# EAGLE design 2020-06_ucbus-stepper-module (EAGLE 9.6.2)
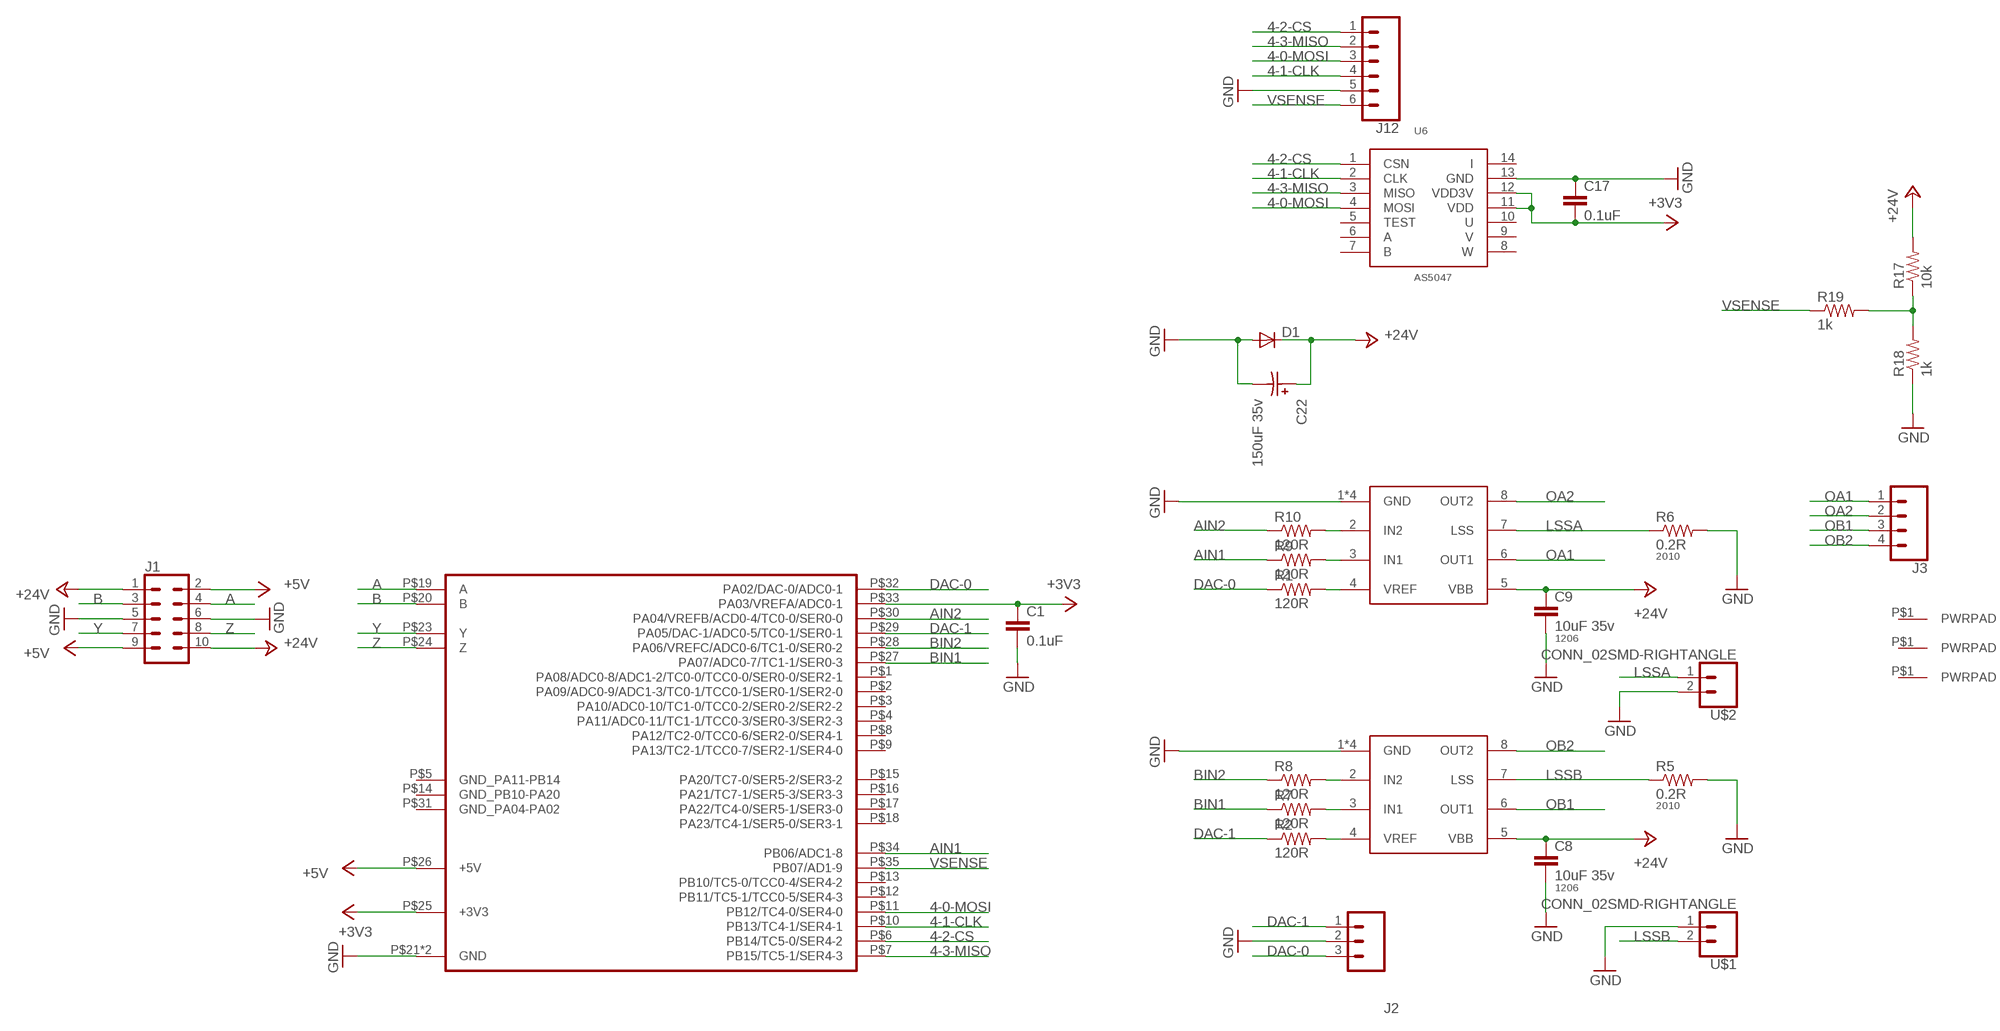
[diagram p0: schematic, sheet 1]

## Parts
C1  0.1uF  CAP0805  [0805]
C8  10uF 35v  CAP1206  [1206]
C9  10uF 35v  CAP1206  [1206]
C17  0.1uF  CAP0805  [0805]
C22  150uF 35v  CAP-POLCAP_POL_SMD6.6X6.6  [SMD-ELEC-CAP]
D1  DIODESMA403D  [SMA-403D]
J1  CONN_05X2SHD_LOCK  [2X5-SHROUDED_LOCK]
J2  CONN_03SMD_RA_MALE  [1X03_SMD_RA_MALE]
J3  CONN_04SCREW_LOCK  [SCREWTERMINAL-3.5MM-4_LOCK]
J4  PWRPADM3-SKINNY  [PWRPAD_3-25MM-SKINNY]
J5  PWRPADM3-SKINNY  [PWRPAD_3-25MM-SKINNY]
J6  PWRPADM3-SKINNY  [PWRPAD_3-25MM-SKINNY]
J12  CONN_06SMD-FEMALE-V2  [1X06-SMD-FEMALE]
R1  120R  RESISTOR0805-RES  [0805]
R2  120R  RESISTOR0805-RES  [0805]
R5  0.2R  RESISTOR2010  [R2010]
R6  0.2R  RESISTOR2010  [R2010]
R7  120R  RESISTOR0805-RES  [0805]
R8  120R  RESISTOR0805-RES  [0805]
R9  120R  RESISTOR0805-RES  [0805]
R10  120R  RESISTOR0805-RES  [0805]
R17  10k  RESISTOR0805-RES  [0805]
R18  1k  RESISTOR0805-RES  [0805]
R19  1k  RESISTOR0805-RES  [0805]
U1  UCBUS_MODULE  [UCBUS_MODULE]
U2  A4950THRU  [SOIC8_PAD_THRU]
U3  A4950THRU  [SOIC8_PAD_THRU]
U6  AS5047  [TSSOP14]
U$1  CONN_02SMD-RIGHTANGLE  [1X02_SMD_RA_MALE]
U$2  CONN_02SMD-RIGHTANGLE  [1X02_SMD_RA_MALE]

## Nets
4-0-MOSI: J12.3 U1.P$11(PB12/TC4-0/SER4-0) U6.4(MOSI)
4-1-CLK: J12.4 U1.P$10(PB13/TC4-1/SER4-1) U6.2(CLK)
4-2-CS: J12.1 U1.P$6(PB14/TC5-0/SER4-2) U6.1(CSN)
4-3-MISO: J12.2 U1.P$7(PB15/TC5-1/SER4-3) U6.3(MISO)
+3V3: C1.1 C17.2 U1.P$25(+3V3) U1.P$33(PA03/VREFA/ADC0-1) U6.11(VDD) U6.12(VDD3V)
+5V: J1.2 J1.9 U1.P$26(+5V)
+24V: C8.1 C9.1 C22.A D1.P$1(C) J1.1 J1.10 R17.2 U2.5(VBB) U3.5(VBB)
A: J1.4 U1.P$19(A)
AIN1: R9.1 U1.P$34(PB06/ADC1-8)
AIN2: R10.1 U1.P$30(PA04/VREFB/ACD0-4/TC0-0/SER0-0)
B: J1.3 U1.P$20(B)
BIN1: R7.1 U1.P$27(PA07/ADC0-7/TC1-1/SER0-3)
BIN2: R8.1 U1.P$28(PA06/VREFC/ADC0-6/TC1-0/SER0-2)
DAC-0: J2.3 R1.1 U1.P$32(PA02/DAC-0/ADC0-1)
DAC-1: J2.1 R2.1 U1.P$29(PA05/DAC-1/ADC0-5/TC0-1/SER0-1)
GND: C1.2 C8.2 C9.2 C17.1 C22.C D1.P$2(A) J1.5 J1.6 J2.2 J12.5 R5.2 R6.2 R18.1 U1.P$21(GND) U1.P$22(GND) U2.1(GND) U2.P$1(GND) U2.P$2(GND) U2.P$3(GND) U3.1(GND) U3.P$1(GND) U3.P$2(GND) U3.P$3(GND) U6.13(GND) U$1.1 U$2.2
LSSA: R6.1 U3.7(LSS) U$2.1
LSSB: R5.1 U2.7(LSS) U$1.2
N$1: R9.2 U3.3(IN1)
N$2: R2.2 U2.4(VREF)
N$3: R1.2 U3.4(VREF)
N$4: R10.2 U3.2(IN2)
N$7: R8.2 U2.2(IN2)
N$8: R7.2 U2.3(IN1)
N$17: R17.1 R18.2 R19.2
OA1: J3.1 U3.6(OUT1)
OA2: J3.2 U3.8(OUT2)
OB1: J3.3 U2.6(OUT1)
OB2: J3.4 U2.8(OUT2)
VSENSE: J12.6 R19.1 U1.P$35(PB07/AD1-9)
Y: J1.7 U1.P$23(Y)
Z: J1.8 U1.P$24(Z)
Unconnected: J4.P$1(PWRPAD) J5.P$1(PWRPAD) J6.P$1(PWRPAD) U1.P$1(PA08/ADC0-8/ADC1-2/TC0-0/TCC0-0/SER0-0/SER2-1) U1.P$2(PA09/ADC0-9/ADC1-3/TC0-1/TCC0-1/SER0-1/SER2-0) U1.P$3(PA10/ADC0-10/TC1-0/TCC0-2/SER0-2/SER2-2) U1.P$4(PA11/ADC0-11/TC1-1/TCC0-3/SER0-3/SER2-3) U1.P$5(GND_PA11-PB14) U1.P$8(PA12/TC2-0/TCC0-6/SER2-0/SER4-1) U1.P$9(PA13/TC2-1/TCC0-7/SER2-1/SER4-0) U1.P$12(PB11/TC5-1/TCC0-5/SER4-3) U1.P$13(PB10/TC5-0/TCC0-4/SER4-2) U1.P$14(GND_PB10-PA20) U1.P$15(PA20/TC7-0/SER5-2/SER3-2) U1.P$16(PA21/TC7-1/SER5-3/SER3-3) U1.P$17(PA22/TC4-0/SER5-1/SER3-0) U1.P$18(PA23/TC4-1/SER5-0/SER3-1) U1.P$31(GND_PA04-PA02) U6.5(TEST) U6.6(A) U6.7(B) U6.8(W) U6.9(V) U6.10(U) U6.14(I)

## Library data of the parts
C1 C17 = passives:CAP: Capacitor; PACKAGE: 0805
C8 C9 = passives:CAP: Capacitor; PACKAGE: 1206
C22 = passives:CAP-POL
D1 = passives:DIODE: DIODE
J1 = SparkFun-Connectors:CONN_05X2: Multi connection point. Often used as Generic Header-pin footprint for 0.1 inch spaced/style header connections For AVR SPI programming port, see special device with nice symbol: "AVR_SPI_PROG_5x2.dev" You can populate with any combo of single row headers, but if you'd like an exact match, check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; PROD_ID: CONN-08671; SF_ID: PRT-08506
J2 = SparkFun-Connectors:CONN_03: Multi connection point. Often used as Generic Header-pin footprint for 0.1 inch spaced/style header connections On any of the 0.1 inch spaced packages, you can populate with these: Break Away Headers - Straight (PRT-00116) Break Away Male Headers - Right Angle (PRT-00553) Female Headers (PRT-00115)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; PROD_ID: CONN-10925
J3 = SparkFun-Connectors:CONN_04: Multi connection point. Often used as Generic Header-pin footprint for 0.1 inch spaced/style header connections On any of the 0.1 inch spaced packages, you can populate with these: Break Away Headers - Straight (PRT-00116) Break Away Male Headers - Right Angle (PRT-00553) Female Headers (PRT-00115)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
J4-J6 = connector:PWRPAD
J12 = SparkFun-Connectors:CONN_06: Multi connection point. Often used as Generic Header-pin footprint for 0.1 inch spaced/style header connections On any of the 0.1 inch spaced packages, you can populate with these: Break Away Headers - Straight (PRT-00116) Break Away Male Headers - Right Angle (PRT-00553) Female Headers (PRT-00115)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; PROD_ID: CONN-09668
R1 R2 R7-R10 R17-R19 = passives:RESISTOR: Resistor; PACKAGE: 0805
R5 R6 = passives:RESISTOR: Resistor; PACKAGE: 2010
U1 = connector:UCBUS_MODULE
U2 U3 = power:A4950
U6 = sensor:AS5047
U$1 U$2 = connector:CONN_02

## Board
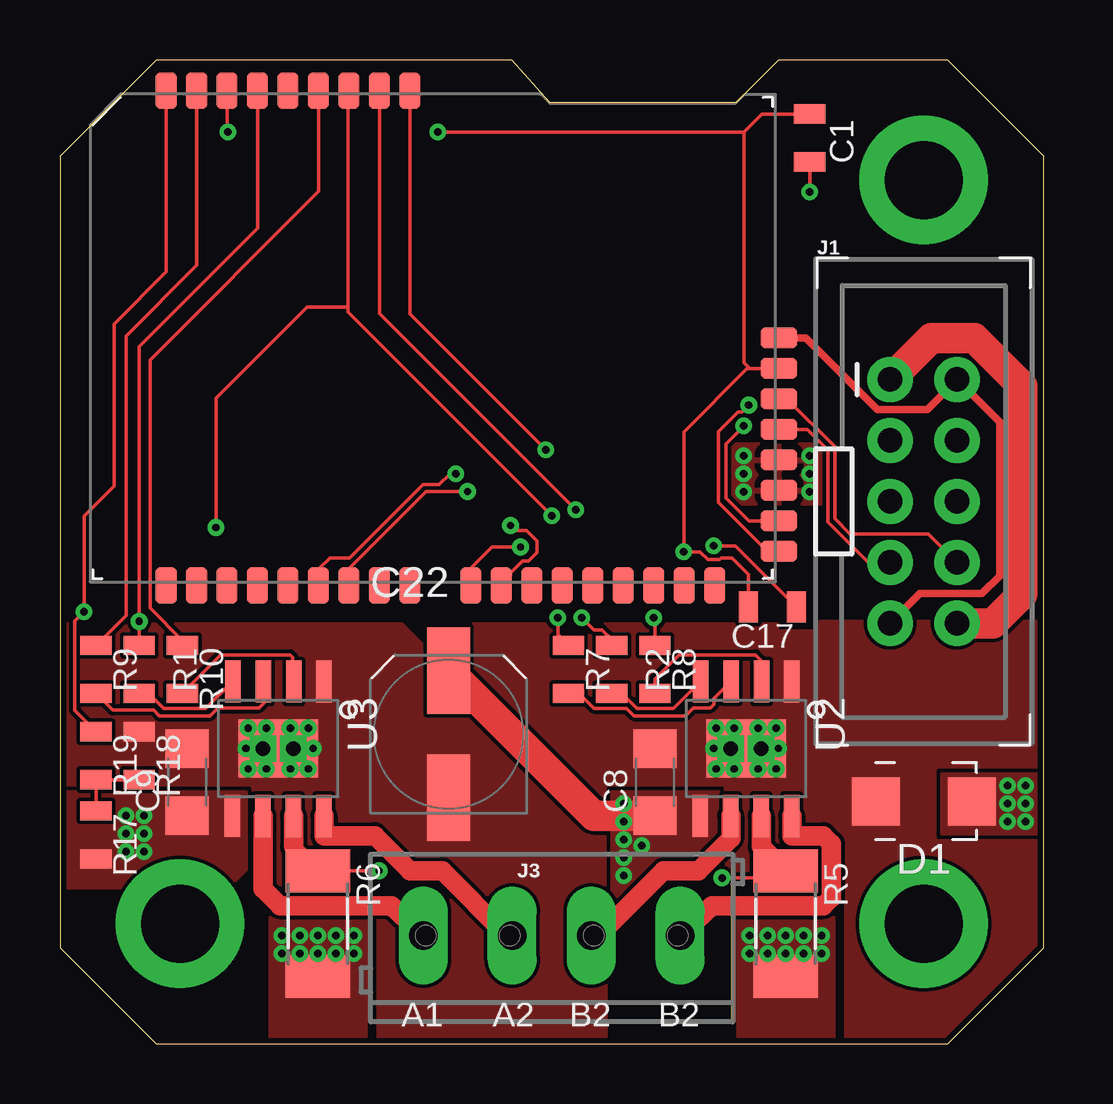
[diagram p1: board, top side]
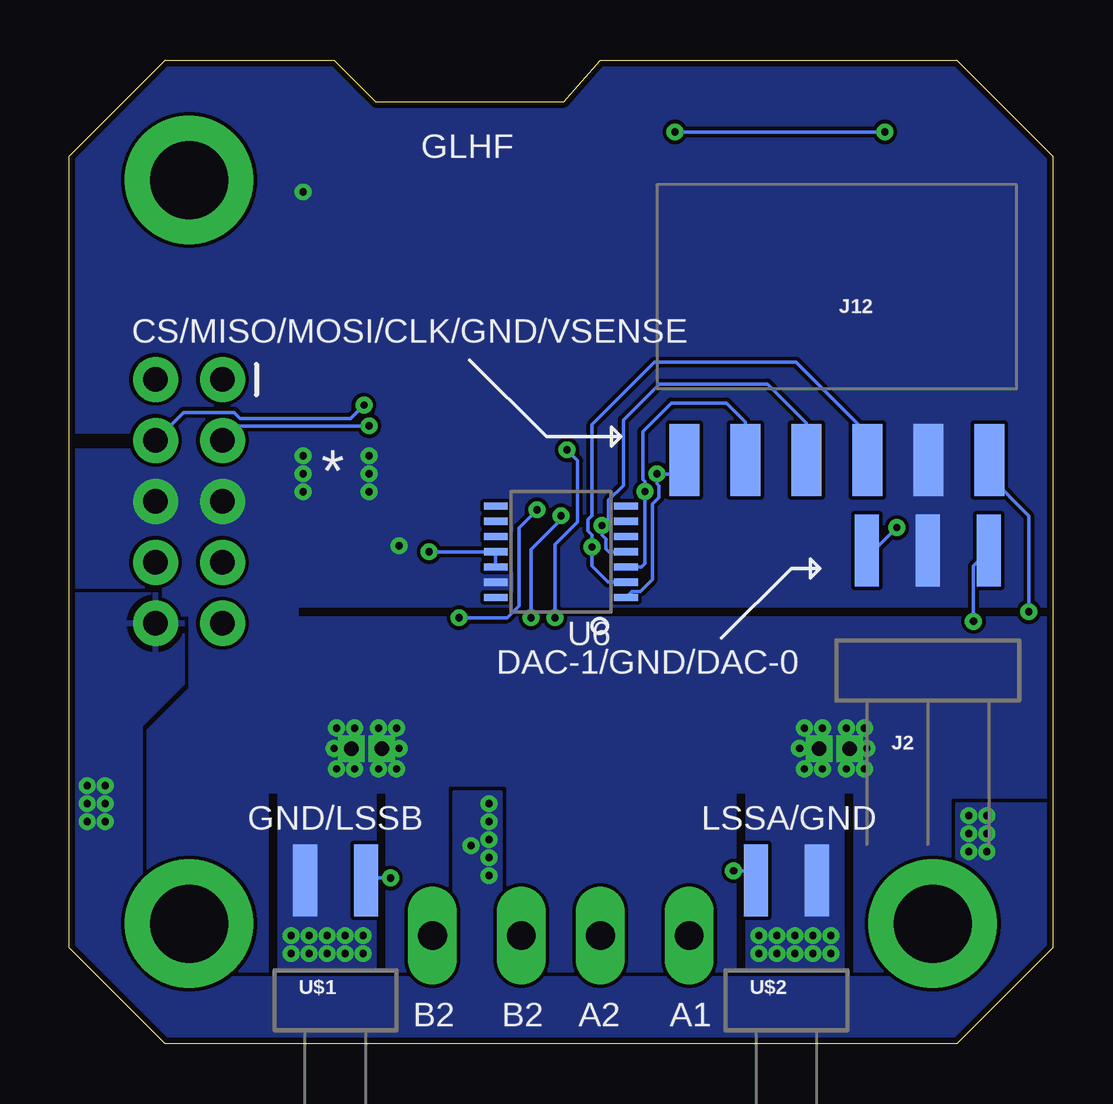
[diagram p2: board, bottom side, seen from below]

Size 41 x 41 mm. Coordinates in mm from the lower left corner, seen from the top.
Outline: 4,0 37,0 41,4 41,37 37,41 29.95,41 28.2,39.25 20.4,39.25 18.85,41 4,41 0,37 0,4 4,0
Copper layers (1*16): Top 0.035mm / dielectric 1.5mm / Bottom 0.035mm
Design rules "default *": minimum track width 6mil, minimum drill 10mil, track to track 6mil, track to pad 6mil, pad to pad 6mil, via to via 6mil, smd to smd 0mil, copper to edge 10mil, drill to drill 6mil, minimum pad ring 10mil, minimum via ring 8mil, stop-mask expansion 4mil, vias tented up to drill 35mil, thermal gap 10mil

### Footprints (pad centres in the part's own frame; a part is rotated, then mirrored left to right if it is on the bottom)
0805 = smd 0.8 x 1.3: 1 -1,0; 2 1,0
1206 = smd 1.6 x 1.8: 1 -1.4,0; 2 1.4,0
SMD-ELEC-CAP = smd 1.8 x 3.6: A 0,2.65; C 0,-2.65
SMA-403D = smd 2 x 2: P$1 -2,0; P$2 2,0
2X5-SHROUDED_LOCK = drill 1.016 pad 1.88: 1 -1.397,5.08; 2 1.397,5.08; 3 -1.397,2.54; 4 1.397,2.54; 5 -1.397,0; 6 1.397,0; 7 -1.397,-2.54; 8 1.397,-2.54; 9 -1.397,-5.08; 10 1.397,-5.08
1X03_SMD_RA_MALE = smd 1 x 3: 1 -2.54,5; 2 0,5; 3 2.54,5
SCREWTERMINAL-3.5MM-4_LOCK = drill 1.2 pad 2.032 long: 1 -0.1,0; 2 3.6,0; 3 6.9,0; 4 10.6,0
PWRPAD_3-25MM-SKINNY = drill 3.25 pad 5.35: P$1 0,0
1X06-SMD-FEMALE = smd 1.25 x 3: 1 6.35,3.425; 2 3.81,3.425; 3 1.27,3.425; 4 -1.27,3.425; 5 -3.81,3.425; 6 -6.35,3.425
R2010 = smd 1.8 x 2.7: 1 -2.2,0; 2 2.2,0
UCBUS_MODULE = smd 0.889 x 1.524: P$1 3.175,-0.152; P$2 4.445,-0.152; P$3 5.715,-0.152; P$4 6.985,-0.152; P$5 8.255,-0.152; P$6 9.525,-0.152; P$7 10.795,-0.152; P$8 12.065,-0.152; P$9 13.335,-0.152; P$10 15.875,-0.152; P$11 17.145,-0.152; P$12 18.415,-0.152; P$13 19.685,-0.152; P$14 20.955,-0.152; P$15 22.225,-0.152; P$16 23.495,-0.152; P$17 24.765,-0.152; P$18 26.035,-0.152; P$27 13.335,20.472; P$28 12.065,20.472; P$29 10.795,20.472; P$30 9.525,20.472; P$31 8.255,20.472; P$32 6.985,20.472; P$33 5.715,20.472; P$34 4.445,20.472; P$35 3.175,20.472 | smd 1.524 x 0.889: P$19 28.727,1.27; P$20 28.727,2.54; P$21 28.727,3.81; P$22 28.727,5.08; P$23 28.727,6.35; P$24 28.727,7.62; P$25 28.727,8.89; P$26 28.727,10.16
SOIC8_PAD_THRU = smd 1.75 x 0.65: 1 -2.8,1.905; 2 -2.8,0.645; 3 -2.8,-0.625; 4 -2.8,-1.895; 5 2.8,-1.905; 6 2.8,-0.635; 7 2.8,0.635; 8 2.8,1.905 | smd 2.41 x 3.3: P$1 0,0 | drill 0.6 square: P$2 0,0.635; P$3 0,-0.635
TSSOP14 = smd 0.305 x 0.991: 1 -1.905,-2.718; 2 -1.27,-2.718; 3 -0.635,-2.718; 4 0,-2.718; 5 0.635,-2.718; 6 1.27,-2.718; 7 1.905,-2.718; 8 1.905,2.718; 9 1.27,2.718; 10 0.635,2.718; 11 0,2.718; 12 -0.635,2.718; 13 -1.27,2.718; 14 -1.905,2.718
1X02_SMD_RA_MALE = smd 1 x 3: 1 -1.27,5; 2 1.27,5

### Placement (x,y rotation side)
C1  31.25,37.75 270 top
C8  24.8,10.9 90 top
C9  5.3,10.9 90 top
C17  29.7,18.2 180 top
C22  16.2,12.9 0 top
D1  36,10.1 180 top
J1  36,22.6 0 top
J2  5.2,15.55 0 bottom
J3  15.25,4.5 0 top
J4  36,5 0 top
J5  36,36 0 top
J6  5,5 0 top
J12  9,27.75 180 bottom
R1  3.3,15.6 270 top
R2  23,15.6 270 top
R5  30.25,5 270 top
R6  10.75,5 270 top
R7  21.2,15.6 270 top
R8  24.8,15.6 270 top
R9  1.5,15.6 270 top
R10  5.1,15.6 270 top
R17  1.5,8.7 270 top
R18  3.3,12 270 top
R19  1.5,12 270 top
U1  1.25,19.25 0 top
U2  28.6,12.3 270 top
U3  9.1,12.3 270 top
U6  20.5,20.5 90 bottom
U$1  29.9,1.8 0 bottom
U$2  11.1,1.8 0 bottom

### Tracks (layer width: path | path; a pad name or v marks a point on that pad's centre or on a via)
4-0-MOSI  (via drill 0.3)
  Top 0.152: U1.P$11 18.78,19.49 18.78,19.61 19.29,20.12 19.54,20.12 19.88,20.46 19.88,20.94 19.44,21.38 19,21.38 v18.78,21.6
  Bottom 0.152: U6.4 18.5,20.5 18.62,20.62 18.62,21.04 18.78,21.21 v18.78,21.6 18.51,21.88 18.51,22.65 17.9,23.26 17.9,26 16.4,27.5 11.9,27.5 10.27,25.87 J12.3
4-1-CLK  (via drill 0.3)
  Top 0.152: v19.2,20.7 18,20.7 17.12,19.82 U1.P$10
  Bottom 0.152: U6.2 18.53,19.23 19.2,19.9 v19.2,20.7 19.2,21.19 19.36,21.36 19.36,21.84 19.2,22 19.2,25.8 16.6,28.4 10.7,28.4 7.73,25.43 J12.4
4-2-CS  (via drill 0.3)
  Top 0.152: v16.5,23.75 16.25,23.75 15.81,23.31 15.13,23.31 12.07,20.25 11.25,20.25 10.78,19.77 U1.P$6
  Bottom 0.152: U6.1 17.53,18.85 17.19,18.85 16.69,19.35 16.69,22.49 16.41,22.77 16.41,23.25 16.5,23.34 v16.5,23.75 15.93,23.75 J12.1
4-3-MISO  (via drill 0.3)
  Top 0.152: v16.99,23.01 15.26,23.01 12.04,19.8 U1.P$7
  Bottom 0.152: U6.3 17.14,19.86 16.99,20.01 v16.99,23.01 16.99,23.42 17.08,23.51 17.08,25.52 15.9,26.7 13.6,26.7 12.81,25.91 J12.2
+3V3  (via drill 0.3)
  Top 0.152: C17.2 28.7,19.55 28,20.25 27.57,20.25 27.49,20.17 27.01,20.17 26.68,20.5 v26,20.5 26,25.5 28.64,28.14 28.75,28.14 | U1.P$25 28.75,28.14 | U1.P$33 6.96,38.03 v7,38 | v15.75,38 28.5,38 | 28.5,38 29.25,38.75 C1.1 | 28.75,28.14 28.5,28.39 28.5,38
  Bottom 0.152: U6.12 U6.11 v26,20.5 | v7,38 v15.75,38
+5V
  Top 0.305: J1.9 35.85,18.77 38.44,18.77 39.17,19.5 39.17,25.91 J1.2 36.15,26.43 34.06,26.43 31.09,29.41 U1.P$26
+24V  (via drill 0.3)
  Top 1.27: J1.1 36.33,29.41 38.11,29.41 40.11,27.41 40.11,18.75 38.88,17.52 J1.10 | C22.A 22.25,9.5 C8.1
  other vias: 2.75,9.5 2.75,8.75 2.75,8 3.5,8 3.5,8.75 3.5,9.5 23.5,10 23.5,9.25 23.5,8.5 23.5,7.75 23.5,7 24.25,8.25 39.5,10.75 39.5,10 39.5,9.25 40.25,9.25 40.25,10 40.25,10.75
  pour Bottom: 36.25,18.75 36.25,15 38,13.25 38,5.75 35,2.75 24.95,2.75 24.95,10.5 23,10.5 23,2.75 6,2.75 4,4.75 4,10 -2,10 -2,-2 42.5,-2 42.5,18.75
  pour Top (no thermals): 7.75,10.5 7.75,7.25 7,6.5 -0.5,6.5 -0.5,10.5
  pour Top (no thermals): 23,10.5 27.25,10.5 27.5,10.5 27.5,7.5 25.25,7.5 23.5,5.75 23,5.75
  pour Top (no thermals): 36.75,11.25 43,11.25 43,8.75 36.75,8.75
A  (via drill 0.3)
  Top 0.152: U1.P$19 29.48,20.52 27.45,22.55 27.45,25.52 28.26,26.33 28.43,26.33 v28.71,26.61
  Bottom 0.152: v28.71,26.61 29.26,26.05 33.87,26.05 34.12,26.31 36.23,26.31 J1.4
AIN1
  Top 0.152: R9.1 2.75,17.85 2.75,29.5 5.7,32.45 U1.P$34
AIN2
  Top 0.152: R10.1 5.1,16.8 3.75,18.15 3.75,28.5 10.78,35.52 U1.P$30
B  (via drill 0.3)
  Top 0.152: U1.P$20 28.71,21.79 27.75,22.75 27.75,25 v28.5,25.75
  Bottom 0.152: v28.5,25.75 33.99,25.75 J1.3
BIN1  (via drill 0.3)
  Top 0.152: v20.75,17.75 20.75,17.05 R7.1 | v20.25,24.75 14.59,30.41 U1.P$27
  Bottom 0.152: v20.75,17.75 20.75,20.8 19.8,21.75 19.8,24.3 v20.25,24.75
BIN2  (via drill 0.3)
  Top 0.152: R8.1 24.8,17.7 v24.75,17.75 | U1.P$28 13.31,30.43 v21.5,22.25
  Bottom 0.152: v24.75,17.75 22.75,17.75 22.25,18.25 22.25,21.5 v21.5,22.25
DAC-0  (via drill 0.3)
  Top 0.152: R1.1 v3.3,17.6 3.3,29.05 8.23,33.98 U1.P$32
  Bottom 0.152: J2.3 3.3,19.91 v3.3,17.6
DAC-1  (via drill 0.3)
  Top 0.152: v21.75,17.75 22.25,17.25 22.6,17.25 23,16.85 R2.1 | v20.5,22 12,30.5 12,30.7 | 12,30.7 12,39.68 U1.P$29 | 12,30.7 10.3,30.7 6.5,26.9 v6.5,21.5
  Bottom 0.152: v20.5,22 20.5,21.85 21.75,20.6 v21.75,17.75 | v6.5,21.5 7.46,20.55 J2.1
GND  (via drill 0.3)
  Top 0.152: C17.1 28.15,20.75 v27.25,20.75 | C1.2 v31.25,35.5
  other vias: 29.85,13.15 9.25,4.5 10,4.5 10.75,4.5 11.5,4.5 12.25,4.5 9.25,3.75 10,3.75 10.75,3.75 11.5,3.75 12.25,3.75 28.75,4.5 29.5,4.5 30.25,4.5 31,4.5 31.75,4.5 28.75,3.75 29.5,3.75 30.25,3.75 31,3.75 31.75,3.75 29.1,13.15 28.1,13.15 27.35,13.15 29.1,11.45 29.85,11.45 29.95,12.3 27.25,12.3 27.35,11.45 28.1,11.45 10.35,13.15 9.6,13.15 8.6,13.15 7.85,13.15 9.6,11.45 10.35,11.45 10.55,12.3 7.75,12.3 7.85,11.45 8.6,11.45 28.5,24.5 28.5,23.75 28.5,23 31.25,24.5 31.25,23.75 31.25,23
  pour Bottom (rank 4, no thermals): 41.5,41.5 41.5,25.5 38,25.5 38,24.75 41.5,24.75 41.5,-0.5 32.75,-0.5 32.75,10.5 32.25,10.5 32.25,-0.5 28.25,-0.5 28.25,10.5 27.75,10.5 27.75,-0.5 13.25,-0.5 13.25,10.5 12.75,10.5 12.75,-0.5 8.75,-0.5 8.75,10.5 8.25,10.5 8.25,-0.5 -1,-0.5 -1,17.75 31.5,17.75 31.5,18.25 -1,18.25 -1,41.5
  pour Top (rank 4, no thermals): 8.75,-1.5 8.75,5.25 12.75,5.25 12.75,-1.5
  pour Top (rank 4, no thermals): 28.25,-1.25 28.25,5.25 32.25,5.25 32.25,-1.25
  pour Top (rank 4, no thermals): 29.9,17.5 29.9,17.2 31.7,17.2 31.7,17.6 41.9,17.6 42,17.5 42,-1.25 32.75,-1.25 32.75,6.25 27.75,6.25 27.75,-1.25 23.25,-1.25 23.25,9.25 15,17.5
  pour Top (rank 4, no thermals): -1.5,17.5 -1.5,-1.5 8.25,-1.5 8.25,6.25 13.25,6.25 13.25,-1.5 22.75,-1.5 22.75,9 14.25,17.5
  pour Top: 28,25 31.75,25 31.75,22.5 28,22.5
LSSA  (via drill 0.3)
  Top 0.152: R6.1 v13.3,7.2
  Top 0.61: 9.73,8.21 R6.1
  Top 0.813: U3.7 9.73,8.21
  Bottom 0.152: U$2.1 12.77,7.2 v13.3,7.2
LSSB  (via drill 0.3)
  Top 0.152: R5.1 29.95,6.9 v27.6,6.9
  Top 0.813: U2.7 29.23,8.21 R5.1
  Bottom 0.152: v27.6,6.9 28.53,6.9 U$1.2
N$1
  Top 0.152: R9.2 2.2,13.9 3.9,13.9 4.13,13.67 6.27,13.67 6.6,14 8.3,14 8.5,14.2 8.5,15.07 U3.3
N$2
  Top 0.152: R2.2 23.43,14.6 24.05,13.97 25.58,13.97 U2.4
N$3
  Top 0.152: R1.2 3.7,14.6 4.33,13.97 6.08,13.97 U3.4
N$4
  Top 0.152: U3.2 9.7,15.14 9.7,16.1 9.6,16.2 8.9,16.2 8.89,16.2 6.7,16.2 R10.2
N$7
  Top 0.152: R8.2 24.8,15.2 25.8,16.2 29,16.2 29.25,15.96 U2.2
N$8
  Top 0.152: R7.2 21.63,14.6 22.25,13.97 23.62,13.97 23.93,13.67 26.07,13.67 26.4,14 27.12,14 27.26,14.13 27.26,14.38 U2.3
N$17
  Top 0.152: R17.1 R19.2 R18.2
OA1
  Top 0.813: J3.1 13.83,5.74 9.17,5.74 8.46,6.45 U3.6
OA2
  Top 0.813: J3.2 18.64,4.5 15.94,7.21 14.58,7.21 13.13,8.66 11,8.66 11.01,8.66 U3.8
OB1
  Top 0.813: J3.3 22.45,4.5 25.16,7.21 26.62,7.21 27.96,8.55 U2.6
OB2
  Top 0.813: J3.4 27.17,5.74 31.83,5.74 32.16,6.07 32.16,8.33 31.83,8.66 30.5,8.66 U2.8
VSENSE  (via drill 0.3)
  Top 0.152: R19.1 0.62,13.88 0.62,17.62 v1,18 1,22 2.25,23.25 2.25,30 4.42,32.17 U1.P$35
  Bottom 0.152: J12.6 2.65,23.65 1,22 v1,18
Y
  Top 0.152: U1.P$23 31.15,25.6 32,24.75 32,21.75 33.69,20.06 J1.7
Z
  Top 0.152: U1.P$24 30.31,26.87 32.3,24.88 32.3,21.88 32.93,21.25 36.21,21.25 J1.8

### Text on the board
tPlace: A1 | A2 | B2 | B2
bPlace: GLHF | CS/MISO/MOSI/CLK/GND/VSENSE | * | DAC-1/GND/DAC-0 | LSSA/GND | GND/LSSB | A1 | A2 | B2 | B2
